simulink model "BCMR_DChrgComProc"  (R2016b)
settings: Solver=FixedStepDiscrete  StartTime=0.0  StopTime=10.0  FixedStep=0.01  RelTol=1e-3  EnableMultiTasking=on
undefined symbols (not defined in the file or in its folder): BCMR_ahBattRatdCpctyBrm_C, BCMR_BattSocErrBsmEna_C, BCMR_eBattRatedEnrgBcp_C, BCMR_G1E0PlatformSwCom_C, BCMR_iMaxChrgCurrPmtdBcp_C, BCMR_numBattTypeBrm_C, BCMR_numComVer2011Brm_C, BCMR_numComVer2015Brm_C, BCMR_tMaxTempPmtdBcp_C, BCMR_uBattRatdPackVoltBcp_C, BCMR_uBattRatdPackVoltBrm_C, BCMR_uMaxChrgCellVoltPmtdBcp_C, BCMR_uMaxPmtDChrgVolt_C
libraries: simulink x32
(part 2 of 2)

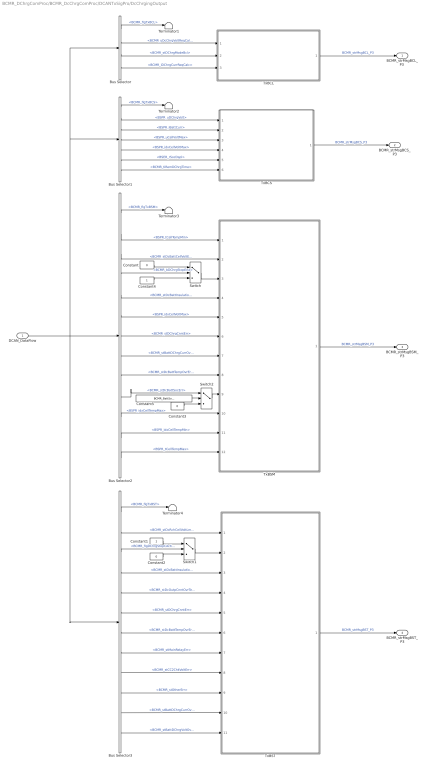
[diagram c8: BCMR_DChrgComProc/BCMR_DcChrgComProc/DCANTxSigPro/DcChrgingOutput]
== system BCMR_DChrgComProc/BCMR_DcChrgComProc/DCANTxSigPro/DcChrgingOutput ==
  DCAN_DataFlow : Inport
  Bus Selector : BusSelector  OutputSignals=BCMR_flgTxBCL,BCMR_uDcChrgVoltReqCalc,BCMR_stDChrgModeBcl,BCMR_iDChrgCurrReqCalc
  Bus Selector1 : BusSelector  OutputSignals=BCMR_flgTxBCS,BSPR_uDChrgVolt,BSPR_iBattCurr,BSPR_uCellVoltMax,BSPR_idxCellVoltMax,BSER_rSocDspl,BCMR_tiRemDChrgTime
  Bus Selector2 : BusSelector  OutputSignals=BCMR_flgTxBSM,BSPR_tCellTempMin,BCMR_stDcBattCellVoltErr,BCMR_bDChrgStopEna,BCMR_stDcBattInsulationErr,BSPR_idxCellVoltMax,BCMR_stDChrgCnntErr,BCMR_stBattDChrgCurrOvrErr,BCMR_stDcBattTempOvrErr,BCMR_stDcBattSocErr,BSPR_idxCellTempMax,BSPR_idxCellTempMin,BSPR_tCellTempMax
  Bus Selector3 : BusSelector  OutputSignals=BCMR_flgTxBST,BCMR_stDcRchCellVoltLmt,BCMR_flgDChrgStopCActive,BCMR_stDcBattInsulationErr,BCMR_stDcOutpCnntOvrTempErr,BCMR_stDChrgCnntErr,BCMR_stDcBattTempOvrErr,BCMR_stMainRelayErr,BCMR_stCC2ChkVoltErr,BCMR_stOtherErr,BCMR_stBattDChrgCurrOvrErr,BCMR_stBattDChrgVoltOvrErr
  Constant : Constant  Value=0  OutDataTypeStr=uint8
  Constant1 : Constant  OutDataTypeStr=uint8
  Constant2 : Constant  Value=0  OutDataTypeStr=uint8
  Constant3 : Constant  Value=0  OutDataTypeStr=uint8
  Constant4 : Constant  OutDataTypeStr=uint8
  Constant5 : Constant  Value=BCMR_BattSocErrBsmEna_C
  Switch : Switch  Criteria=u2 > Threshold  OutDataTypeStr=uint8
  Switch1 : Switch  Criteria=u2 > Threshold  OutDataTypeStr=uint8
  Switch2 : Switch  Criteria=u2 > Threshold  OutDataTypeStr=uint8
  Terminator{1..4} (4 alike) : Terminator
  TxBCL : Subsystem
  TxBCS : Subsystem
  TxBSM : Subsystem
  TxBST : Subsystem
  "BCMR_strMsgBCL_P3 " : Outport  OutDataTypeStr=Bus: MSG_BCL_P3
  BCMR_strMsgBCS_P3 : Outport  Port=2  OutDataTypeStr=Bus: MSG_BCS_P3
  BCMR_strMsgBSM_P3 : Outport  Port=3  OutDataTypeStr=Bus: MSG_BSM_P3
  BCMR_strMsgBST_P3 : Outport  Port=4  OutDataTypeStr=Bus: MSG_BST_P3
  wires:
  TxBCL/1("BCMR_strMsgBCL_P3 ") -> "BCMR_strMsgBCL_P3 "/1  "BCMR_strMsgBCL_P3"
  TxBCS/1(BCMR_strMsgBCS_P3) -> BCMR_strMsgBCS_P3/1  "BCMR_strMsgBCS_P3"
  TxBSM/1(BCMR_strMsgBSM_P3) -> BCMR_strMsgBSM_P3/1  "BCMR_strMsgBSM_P3"
  DCAN_DataFlow/1 -> Bus Selector/1, Bus Selector1/1, Bus Selector3/1, Bus Selector2/1
  Bus Selector2/2 -> TxBSM/1(BCMR_tBattMinTempBsm)  "<BSPR_tCellTempMin>"
  Bus Selector2/3 -> TxBSM/2(BCMR_stBattCellVoltErrBsm)  "<BCMR_stDcBattCellVoltErr>"
  Bus Selector2/5 -> TxBSM/4(BCMR_stBattInsulationErrBsm)  "<BCMR_stDcBattInsulationErr>"
  Bus Selector2/6 -> TxBSM/5(BCMR_numMaxCellVoltAddrBsm)  "<BSPR_idxCellVoltMax>"
  Bus Selector2/7 -> TxBSM/6(BCMR_stBattOutputContErrBsm)  "<BCMR_stDChrgCnntErr>"
  Bus Selector2/8 -> TxBSM/7(BCMR_stBattChrgCurrOvrErrBsm)  "<BCMR_stBattDChrgCurrOvrErr>"
  Bus Selector2/9 -> TxBSM/8(BCMR_stBattTempOvrErrBsm)  "<BCMR_stDcBattTempOvrErr>"
  TxBST/1(BCMR_strMsgBST_P3) -> BCMR_strMsgBST_P3/1  "BCMR_strMsgBST_P3"
  Bus Selector/2 -> TxBCL/1(BCMR_vDcChrgVoltReqBcl)  "<BCMR_uDcChrgVoltReqCalc>"
  Bus Selector/3 -> TxBCL/2(BCMR_stDcChrgModeBcl)  "<BCMR_stDChrgModeBcl>"
  Bus Selector/4 -> TxBCL/3(BCMR_iDcChrgCurrReqBcl)  "<BCMR_iDChrgCurrReqCalc>"
  Bus Selector1/2 -> TxBCS/1(BCMR_vDcChrgVoltReqBcs)  "<BSPR_uDChrgVolt>"
  Bus Selector1/3 -> TxBCS/2(BCMR_iDcChrgCurrReqBcs)  "<BSPR_iBattCurr>"
  Bus Selector1/4 -> TxBCS/3(BCMR_uMaxCellVoltBcs)  "<BSPR_uCellVoltMax>"
  Bus Selector1/5 -> TxBCS/4(BCMR_numMaxCellVoltGrpNumBcs)  "<BSPR_idxCellVoltMax>"
  Bus Selector1/6 -> TxBCS/5(BCMR_rSocDsplBcs)  "<BSER_rSocDspl>"
  Bus Selector1/7 -> TxBCS/6(BCMR_tiDcChrgRemTimeBcs)  "<BCMR_tiRemDChrgTime>"
  Bus Selector2/11 -> TxBSM/10(BCMR_numBattMaxTemptAddrBsm)  "<BSPR_idxCellTempMax>"
  Bus Selector2/12 -> TxBSM/11(BCMR_numBattMinTemptAddrBsm)  "<BSPR_idxCellTempMin>"
  Bus Selector2/13 -> TxBSM/12(BCMR_tBattMaxTempBsm)  "<BSPR_tCellTempMax>"
  Bus Selector3/2 -> TxBST/1(BCMR_stRchCellVoltLmtBst)  "<BCMR_stDcRchCellVoltLmt>"
  Bus Selector3/4 -> TxBST/3(BCMR_stBattInsulationErrBst)  "<BCMR_stDcBattInsulationErr>"
  Bus Selector3/5 -> TxBST/4(BCMR_stOutpCnntOvrTempErrBst)  "<BCMR_stDcOutpCnntOvrTempErr>"
  Bus Selector3/6 -> TxBST/5(BCMR_stChrgCnntErrBst)  "<BCMR_stDChrgCnntErr>"
  Bus Selector3/7 -> TxBST/6(BCMR_stBattOvrTempErrBst)  "<BCMR_stDcBattTempOvrErr>"
  Bus Selector3/8 -> TxBST/7(BCMR_stMainRelayErrBst)  "<BCMR_stMainRelayErr>"
  Bus Selector3/9 -> TxBST/8(BCMR_stCC2ChkVoltErrBst)  "<BCMR_stCC2ChkVoltErr>"
  Bus Selector3/10 -> TxBST/9(BCMR_stOtherErrBst)  "<BCMR_stOtherErr>"
  Bus Selector3/11 -> TxBST/10(BCMR_stChrgCurrAbnrmBst)  "<BCMR_stBattDChrgCurrOvrErr>"
  Bus Selector3/12 -> TxBST/11(BCMR_stChrgVoltAbnrm)  "<BCMR_stBattDChrgVoltOvrErr>"
  Constant/1 -> Switch/1
  Constant4/1 -> Switch/3
  Switch/1 -> TxBSM/3(BCMR_stChrgEnaBsm)
  Bus Selector2/4 -> Switch/2  "<BCMR_bDChrgStopEna>"
  Bus Selector/1 -> Terminator1/1  "<BCMR_flgTxBCL>"
  Bus Selector1/1 -> Terminator2/1  "<BCMR_flgTxBCS>"
  Bus Selector2/1 -> Terminator3/1  "<BCMR_flgTxBSM>"
  Bus Selector3/1 -> Terminator4/1  "<BCMR_flgTxBST>"
  Bus Selector3/3 -> Switch1/2  "<BCMR_flgDChrgStopCActive>"
  Switch1/1 -> TxBST/2(BCMR_stChrgerActStopBst)
  Constant1/1 -> Switch1/1
  Constant2/1 -> Switch1/3
  Constant3/1 -> Switch2/3
  Switch2/1 -> TxBSM/9(BCMR_stBattSocErrBsm)
  Bus Selector2/10 -> Switch2/1  "<BCMR_stDcBattSocErr>"
  Constant5/1 -> Switch2/2

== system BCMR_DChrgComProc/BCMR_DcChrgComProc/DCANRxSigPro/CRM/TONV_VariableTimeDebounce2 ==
  note: Turn On Delay Time Deboune
  u : Inport
  T : Inport  Port=2
  dT : Inport  Port=3
  Add : Sum
  Constant1 : Constant  Value=0  OutDataTypeStr=single
  Constant2 : Constant  OutDataTypeStr=uint8
  Constant3 : Constant  Value=0  OutDataTypeStr=uint8
  Delay : Delay  DelayLength=1  InitialCondition=0
  MinMax : MinMax  Inputs=2
  Product : Product  OutMin=[0]  OutMax=[65535]  OutDataTypeStr=single
  Relational Operator : RelationalOperator  Operator=>  OutDataTypeStr=boolean  RndMeth=Simplest
  Switch : Switch  Criteria=u2 ~= 0
  Switch1 : Switch  Criteria=u2 ~= 0
  y : Outport
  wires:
  Switch1/1 -> Product/1
  Constant3/1 -> Switch1/3
  Constant2/1 -> Switch1/1
  u/1 -> Switch1/2, Switch/2
  dT/1 -> Switch/1
  Constant1/1 -> Switch/3
  Add/1 -> Product/2
  Product/1 -> Relational Operator/1, Delay/1
  Switch/1 -> Add/1
  Delay/1 -> MinMax/2
  Relational Operator/1 -> y/1
  T/1 -> MinMax/1, Relational Operator/2
  MinMax/1 -> Add/2

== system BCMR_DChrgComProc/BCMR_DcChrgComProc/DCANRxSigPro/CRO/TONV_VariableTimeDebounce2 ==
  note: Turn On Delay Time Deboune
  u : Inport
  T : Inport  Port=2
  dT : Inport  Port=3
  Add : Sum
  Constant1 : Constant  Value=0  OutDataTypeStr=single
  Constant2 : Constant  OutDataTypeStr=uint8
  Constant3 : Constant  Value=0  OutDataTypeStr=uint8
  Delay : Delay  DelayLength=1  InitialCondition=0
  MinMax : MinMax  Inputs=2
  Product : Product  OutMin=[0]  OutMax=[65535]  OutDataTypeStr=single
  Relational Operator : RelationalOperator  Operator=>  OutDataTypeStr=boolean  RndMeth=Simplest
  Switch : Switch  Criteria=u2 ~= 0
  Switch1 : Switch  Criteria=u2 ~= 0
  y : Outport
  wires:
  Switch1/1 -> Product/1
  Constant3/1 -> Switch1/3
  Constant2/1 -> Switch1/1
  u/1 -> Switch1/2, Switch/2
  dT/1 -> Switch/1
  Constant1/1 -> Switch/3
  Add/1 -> Product/2
  Product/1 -> Relational Operator/1, Delay/1
  Switch/1 -> Add/1
  Delay/1 -> MinMax/2
  Relational Operator/1 -> y/1
  T/1 -> MinMax/1, Relational Operator/2
  MinMax/1 -> Add/2

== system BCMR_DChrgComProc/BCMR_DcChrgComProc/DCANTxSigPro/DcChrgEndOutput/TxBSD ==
  BCMR_tBattMaxTempBsd : Inport
  BCMR_tBattMinTempBsd : Inport  Port=2
  BCMR_vBattMinCellVoltBsd : Inport  Port=3
  BCMR_vBattMaxCellVoltBsd : Inport  Port=4
  BCMR_rBattSocBsd : Inport  Port=5
  Bus Creator : BusCreator  Inputs=5  OutDataTypeStr=Bus: MSG_BSD_P4
  "BCMR_strMsgBSD_P4 " : Outport  OutDataTypeStr=Bus: MSG_BSD_P4
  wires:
  BCMR_tBattMaxTempBsd/1 -> Bus Creator/1
  BCMR_tBattMinTempBsd/1 -> Bus Creator/2
  BCMR_vBattMinCellVoltBsd/1 -> Bus Creator/3
  BCMR_vBattMaxCellVoltBsd/1 -> Bus Creator/4
  BCMR_rBattSocBsd/1 -> Bus Creator/5
  Bus Creator/1 -> "BCMR_strMsgBSD_P4 "/1

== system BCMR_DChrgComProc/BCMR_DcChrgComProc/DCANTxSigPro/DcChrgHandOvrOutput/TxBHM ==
  Bus Creator : BusCreator  Inputs=1  OutDataTypeStr=Bus: MSG_BHM_P1
  Constant : Constant  Value=BCMR_uMaxPmtDChrgVolt_C
  "BCMR_strMsgBHM_P1 " : Outport  OutDataTypeStr=Bus: MSG_BHM_P1  InitialOutput=[421.8]
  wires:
  Bus Creator/1 -> "BCMR_strMsgBHM_P1 "/1  "BCMR_strMsgBHM_P1"
  Constant/1 -> Bus Creator/1

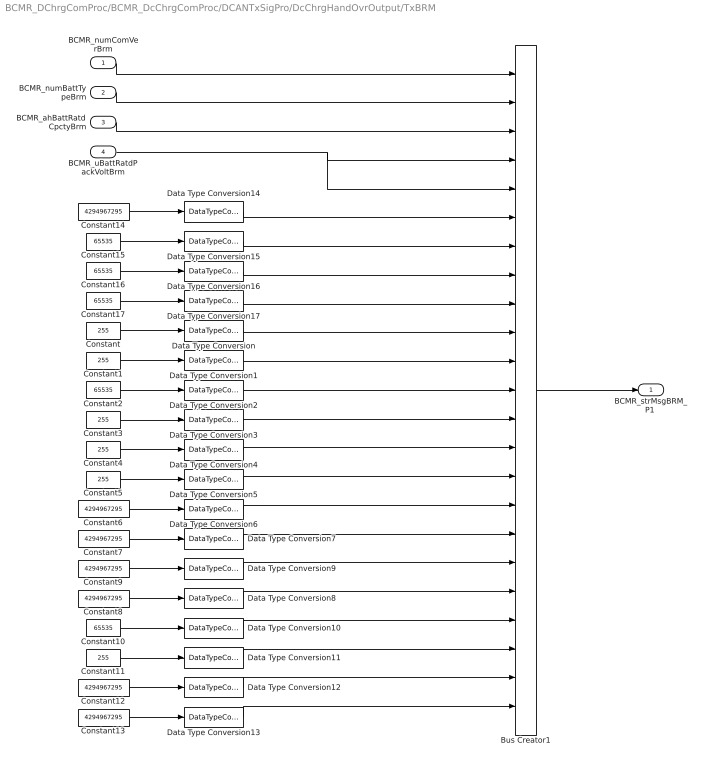
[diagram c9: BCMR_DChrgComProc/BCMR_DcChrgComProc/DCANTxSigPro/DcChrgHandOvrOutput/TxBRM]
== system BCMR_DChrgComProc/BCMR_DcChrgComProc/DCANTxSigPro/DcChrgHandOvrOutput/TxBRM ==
  BCMR_numComVerBrm : Inport
  BCMR_numBattTypeBrm : Inport  Port=2
  BCMR_ahBattRatdCpctyBrm : Inport  Port=3
  BCMR_uBattRatdPackVoltBrm : Inport  Port=4
  Bus Creator1 : BusCreator  Inputs=23  OutDataTypeStr=Bus: MSG_BRM_P1
  Constant{,1,3..5,11} (6 alike) : Constant  Value=255
  Constant{2,10,15..17} (5 alike) : Constant  Value=65535
  Constant{6..9,12..14} (7 alike) : Constant  Value=4294967295
  Data Type Conversion{,1,3..5,11} (6 alike) : DataTypeConversion  OutDataTypeStr=uint8
  Data Type Conversion{2,10,15..17} (5 alike) : DataTypeConversion  OutDataTypeStr=uint16
  Data Type Conversion{6..9,12..14} (7 alike) : DataTypeConversion  OutDataTypeStr=uint32
  "BCMR_strMsgBRM_P1 " : Outport  OutDataTypeStr=Bus: MSG_BRM_P1
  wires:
  BCMR_numBattTypeBrm/1 -> Bus Creator1/2
  BCMR_ahBattRatdCpctyBrm/1 -> Bus Creator1/3
  BCMR_numComVerBrm/1 -> Bus Creator1/1
  Bus Creator1/1 -> "BCMR_strMsgBRM_P1 "/1
  Constant/1 -> Data Type Conversion/1
  Constant1/1 -> Data Type Conversion1/1
  Constant2/1 -> Data Type Conversion2/1
  Constant3/1 -> Data Type Conversion3/1
  Constant4/1 -> Data Type Conversion4/1
  Constant5/1 -> Data Type Conversion5/1
  Constant6/1 -> Data Type Conversion6/1
  Constant7/1 -> Data Type Conversion7/1
  Constant8/1 -> Data Type Conversion8/1
  Constant9/1 -> Data Type Conversion9/1
  Constant10/1 -> Data Type Conversion10/1
  Constant11/1 -> Data Type Conversion11/1
  Constant12/1 -> Data Type Conversion12/1
  Constant13/1 -> Data Type Conversion13/1
  Data Type Conversion13/1 -> Bus Creator1/23
  Data Type Conversion/1 -> Bus Creator1/10
  Data Type Conversion1/1 -> Bus Creator1/11
  Data Type Conversion2/1 -> Bus Creator1/12
  Data Type Conversion3/1 -> Bus Creator1/13
  Data Type Conversion4/1 -> Bus Creator1/14
  Data Type Conversion5/1 -> Bus Creator1/15
  Data Type Conversion6/1 -> Bus Creator1/16
  Data Type Conversion7/1 -> Bus Creator1/17
  Data Type Conversion9/1 -> Bus Creator1/18
  Data Type Conversion8/1 -> Bus Creator1/19
  Data Type Conversion10/1 -> Bus Creator1/20
  Data Type Conversion11/1 -> Bus Creator1/21
  Data Type Conversion12/1 -> Bus Creator1/22
  Constant14/1 -> Data Type Conversion14/1
  Constant15/1 -> Data Type Conversion15/1
  Constant16/1 -> Data Type Conversion16/1
  Constant17/1 -> Data Type Conversion17/1
  Data Type Conversion17/1 -> Bus Creator1/9
  Data Type Conversion14/1 -> Bus Creator1/6
  Data Type Conversion15/1 -> Bus Creator1/7
  Data Type Conversion16/1 -> Bus Creator1/8
  BCMR_uBattRatdPackVoltBrm/1 -> Bus Creator1/5, Bus Creator1/4

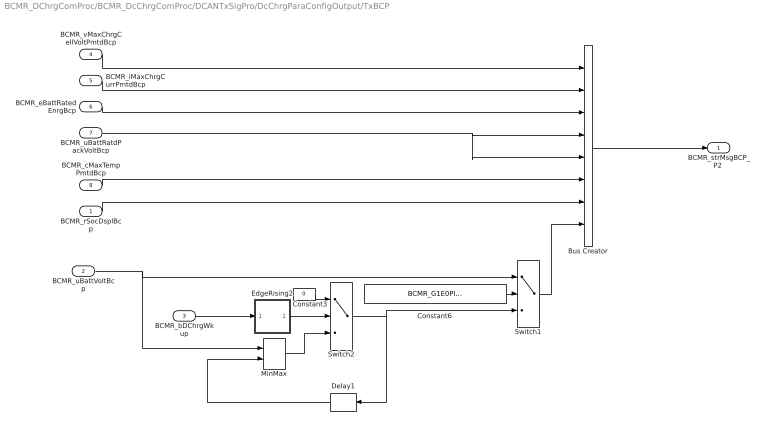
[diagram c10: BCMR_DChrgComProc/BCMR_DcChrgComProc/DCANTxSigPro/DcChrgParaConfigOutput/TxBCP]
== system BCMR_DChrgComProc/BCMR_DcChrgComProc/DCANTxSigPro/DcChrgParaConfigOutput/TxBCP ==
  BCMR_rSocDsplBcp : Inport
  BCMR_uBattVoltBcp : Inport  Port=2
  BCMR_bDChrgWkup : Inport  Port=3
  BCMR_vMaxChrgCellVoltPmtdBcp : Inport  Port=4
  BCMR_iMaxChrgCurrPmtdBcp : Inport  Port=5
  BCMR_eBattRatedEnrgBcp : Inport  Port=6
  BCMR_uBattRatdPackVoltBcp : Inport  Port=7
  BCMR_cMaxTempPmtdBcp : Inport  Port=8
  Bus Creator : BusCreator  Inputs=8  OutDataTypeStr=Bus: MSG_BCP_P2
  Constant3 : Constant  Value=0  OutDataTypeStr=single
  Constant6 : Constant  Value=BCMR_G1E0PlatformSwCom_C
  Delay1 : Delay  DelayLength=1  InitialCondition=0
  EdgeRising2 : Subsystem  TreatAsAtomicUnit=on  RTWFcnName=EdgeRising  RTWFileName=SrvLib
  MinMax : MinMax  Function=max  Inputs=2
  Switch1 : Switch  Criteria=u2 ~= 0
  Switch2 : Switch  Criteria=u2 ~= 0
  "BCMR_strMsgBCP_P2 " : Outport  OutDataTypeStr=Bus: MSG_BCP_P2
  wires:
  BCMR_vMaxChrgCellVoltPmtdBcp/1 -> Bus Creator/1
  BCMR_iMaxChrgCurrPmtdBcp/1 -> Bus Creator/2
  BCMR_eBattRatedEnrgBcp/1 -> Bus Creator/3
  Bus Creator/1 -> "BCMR_strMsgBCP_P2 "/1
  BCMR_rSocDsplBcp/1 -> Bus Creator/7
  BCMR_cMaxTempPmtdBcp/1 -> Bus Creator/6
  BCMR_uBattRatdPackVoltBcp/1 -> Bus Creator/5, Bus Creator/4
  BCMR_bDChrgWkup/1 -> EdgeRising2/1(u)
  EdgeRising2/1(y) -> Switch2/2
  Constant3/1 -> Switch2/1
  Switch2/1 -> Delay1/1, Switch1/3
  MinMax/1 -> Switch2/3
  Delay1/1 -> MinMax/2
  Switch1/1 -> Bus Creator/8
  BCMR_uBattVoltBcp/1 -> Switch1/1, MinMax/1
  Constant6/1 -> Switch1/2

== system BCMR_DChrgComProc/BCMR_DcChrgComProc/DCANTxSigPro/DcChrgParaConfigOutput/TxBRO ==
  BCMR_stBmsRdyBro : Inport
  Bus Creator1 : BusCreator  Inputs=1  OutDataTypeStr=Bus: MSG_BRO_P2
  BCMR_strMsgBRO_P2 : Outport  OutDataTypeStr=Bus: MSG_BRO_P2
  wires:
  BCMR_stBmsRdyBro/1 -> Bus Creator1/1
  Bus Creator1/1 -> BCMR_strMsgBRO_P2/1

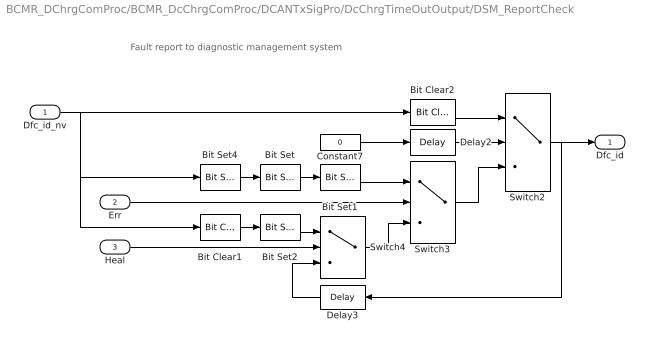
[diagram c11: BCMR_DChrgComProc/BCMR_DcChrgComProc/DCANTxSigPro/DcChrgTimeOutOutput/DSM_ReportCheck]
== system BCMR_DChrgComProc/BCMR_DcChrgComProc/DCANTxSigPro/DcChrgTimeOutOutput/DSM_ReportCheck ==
  note: Fault report to diagnostic management system
  Dfc_id_nv : Inport  OutDataTypeStr=uint8
  Err : Inport  Port=2
  Heal : Inport  Port=3
  Bit Clear1 : simulink/Logic and Bit Operations/Bit Clear  iBit=4
  Bit Clear2 : simulink/Logic and Bit Operations/Bit Clear  iBit=3
  Bit Set : simulink/Logic and Bit Operations/Bit Set  iBit=4
  Bit Set1 : simulink/Logic and Bit Operations/Bit Set  iBit=3
  Bit Set2 : simulink/Logic and Bit Operations/Bit Set  iBit=3
  Bit Set4 : simulink/Logic and Bit Operations/Bit Set  iBit=7
  Constant7 : Constant  Value=0  OutDataTypeStr=boolean
  Delay2 : Delay  DelayLength=1  InitialCondition=1
  Delay3 : Delay  DelayLength=1  InitialCondition=0
  Switch2 : Switch  Criteria=u2 ~= 0
  Switch3 : Switch  Criteria=u2 ~= 0
  Switch4 : Switch  Criteria=u2 ~= 0
  Dfc_id : Outport  OutDataTypeStr=uint8
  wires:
  Dfc_id_nv/1 -> Bit Clear2/1, Bit Set4/1, Bit Clear1/1
  Bit Set4/1 -> Bit Set/1
  Constant7/1 -> Delay2/1
  Delay2/1 -> Switch2/2
  Switch3/1 -> Switch2/3
  Bit Clear2/1 -> Switch2/1
  Switch2/1 -> Delay3/1, Dfc_id/1
  Bit Set1/1 -> Switch3/1
  Bit Set/1 -> Bit Set1/1
  Switch4/1 -> Switch3/3
  Err/1 -> Switch3/2
  Bit Set2/1 -> Switch4/1
  Bit Clear1/1 -> Bit Set2/1
  Delay3/1 -> Switch4/3
  Heal/1 -> Switch4/2

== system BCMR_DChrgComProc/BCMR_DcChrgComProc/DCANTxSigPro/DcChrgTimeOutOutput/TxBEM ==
  BCMR_stSpn3901TimeoutBem : Inport
  BCMR_stSpn3902TimeoutBem : Inport  Port=2
  BCMR_stSpn3903TimeoutBem : Inport  Port=3
  BCMR_stSpn3904TimeoutBem : Inport  Port=4
  BCMR_stSpn3905TimeoutBem : Inport  Port=5
  BCMR_stSpn3906TimeoutBem : Inport  Port=6
  BCMR_stSpn3907TimeoutBem : Inport  Port=7
  BCMR_stOtherErrBem : Inport  Port=8
  Bus Creator : BusCreator  Inputs=8  OutDataTypeStr=Bus: MSG_BEM_ERR
  "BCMR_strMsgBEM_ERR " : Outport  OutDataTypeStr=Bus: MSG_BEM_ERR
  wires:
  Bus Creator/1 -> "BCMR_strMsgBEM_ERR "/1
  BCMR_stSpn3901TimeoutBem/1 -> Bus Creator/1
  BCMR_stSpn3902TimeoutBem/1 -> Bus Creator/2
  BCMR_stSpn3903TimeoutBem/1 -> Bus Creator/3
  BCMR_stSpn3904TimeoutBem/1 -> Bus Creator/4
  BCMR_stSpn3905TimeoutBem/1 -> Bus Creator/5
  BCMR_stSpn3906TimeoutBem/1 -> Bus Creator/6
  BCMR_stSpn3907TimeoutBem/1 -> Bus Creator/7
  BCMR_stOtherErrBem/1 -> Bus Creator/8

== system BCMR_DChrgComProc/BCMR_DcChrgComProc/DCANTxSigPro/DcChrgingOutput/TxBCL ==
  BCMR_vDcChrgVoltReqBcl : Inport
  BCMR_stDcChrgModeBcl : Inport  Port=2
  BCMR_iDcChrgCurrReqBcl : Inport  Port=3
  Bus Creator : BusCreator  Inputs=3  OutDataTypeStr=Bus: MSG_BCL_P3
  Gain : Gain  Gain=-1
  "BCMR_strMsgBCL_P3 " : Outport  OutDataTypeStr=Bus: MSG_BCL_P3
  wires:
  Bus Creator/1 -> "BCMR_strMsgBCL_P3 "/1
  BCMR_iDcChrgCurrReqBcl/1 -> Gain/1
  BCMR_stDcChrgModeBcl/1 -> Bus Creator/2
  BCMR_vDcChrgVoltReqBcl/1 -> Bus Creator/1
  Gain/1 -> Bus Creator/3

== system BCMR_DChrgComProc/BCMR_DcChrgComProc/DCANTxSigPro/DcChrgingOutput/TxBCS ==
  BCMR_vDcChrgVoltReqBcs : Inport
  BCMR_iDcChrgCurrReqBcs : Inport  Port=2
  BCMR_uMaxCellVoltBcs : Inport  Port=3
  BCMR_numMaxCellVoltGrpNumBcs : Inport  Port=4
  BCMR_rSocDsplBcs : Inport  Port=5
  BCMR_tiDcChrgRemTimeBcs : Inport  Port=6
  Bus Creator1 : BusCreator  Inputs=6  OutDataTypeStr=Bus: MSG_BCS_P3
  Data Type Conversion : DataTypeConversion  OutDataTypeStr=uint8
  Data Type Conversion1 : DataTypeConversion  OutDataTypeStr=uint16
  BCMR_strMsgBCS_P3 : Outport  OutDataTypeStr=Bus: MSG_BCS_P3
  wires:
  BCMR_numMaxCellVoltGrpNumBcs/1 -> Bus Creator1/4
  BCMR_uMaxCellVoltBcs/1 -> Bus Creator1/3
  BCMR_iDcChrgCurrReqBcs/1 -> Bus Creator1/2
  BCMR_vDcChrgVoltReqBcs/1 -> Bus Creator1/1
  BCMR_tiDcChrgRemTimeBcs/1 -> Data Type Conversion1/1
  Data Type Conversion/1 -> Bus Creator1/5
  Data Type Conversion1/1 -> Bus Creator1/6
  Bus Creator1/1 -> BCMR_strMsgBCS_P3/1
  BCMR_rSocDsplBcs/1 -> Data Type Conversion/1

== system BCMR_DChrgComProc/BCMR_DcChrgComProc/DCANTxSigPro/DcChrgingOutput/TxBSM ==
  BCMR_tBattMinTempBsm : Inport
  BCMR_stBattCellVoltErrBsm : Inport  Port=2
  BCMR_stChrgEnaBsm : Inport  Port=3
  BCMR_stBattInsulationErrBsm : Inport  Port=4
  BCMR_numMaxCellVoltAddrBsm : Inport  Port=5
  BCMR_stBattOutputContErrBsm : Inport  Port=6
  BCMR_stBattChrgCurrOvrErrBsm : Inport  Port=7
  BCMR_stBattTempOvrErrBsm : Inport  Port=8
  BCMR_stBattSocErrBsm : Inport  Port=9
  BCMR_numBattMaxTemptAddrBsm : Inport  Port=10
  BCMR_numBattMinTemptAddrBsm : Inport  Port=11
  BCMR_tBattMaxTempBsm : Inport  Port=12
  Bus Creator2 : BusCreator  Inputs=12  OutDataTypeStr=Bus: MSG_BSM_P3
  BCMR_strMsgBSM_P3 : Outport  OutDataTypeStr=Bus: MSG_BSM_P3
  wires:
  BCMR_stBattTempOvrErrBsm/1 -> Bus Creator2/8
  BCMR_stBattChrgCurrOvrErrBsm/1 -> Bus Creator2/7
  BCMR_stBattOutputContErrBsm/1 -> Bus Creator2/6
  BCMR_numMaxCellVoltAddrBsm/1 -> Bus Creator2/5
  BCMR_stBattInsulationErrBsm/1 -> Bus Creator2/4
  BCMR_stBattCellVoltErrBsm/1 -> Bus Creator2/2
  BCMR_tBattMinTempBsm/1 -> Bus Creator2/1
  BCMR_stBattSocErrBsm/1 -> Bus Creator2/9
  BCMR_numBattMaxTemptAddrBsm/1 -> Bus Creator2/10
  BCMR_numBattMinTemptAddrBsm/1 -> Bus Creator2/11
  BCMR_tBattMaxTempBsm/1 -> Bus Creator2/12
  BCMR_stChrgEnaBsm/1 -> Bus Creator2/3
  Bus Creator2/1 -> BCMR_strMsgBSM_P3/1

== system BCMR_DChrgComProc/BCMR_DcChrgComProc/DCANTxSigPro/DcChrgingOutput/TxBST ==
  BCMR_stRchCellVoltLmtBst : Inport
  BCMR_stChrgerActStopBst : Inport  Port=2
  BCMR_stBattInsulationErrBst : Inport  Port=3
  BCMR_stOutpCnntOvrTempErrBst : Inport  Port=4
  BCMR_stChrgCnntErrBst : Inport  Port=5
  BCMR_stBattOvrTempErrBst : Inport  Port=6
  BCMR_stMainRelayErrBst : Inport  Port=7
  BCMR_stCC2ChkVoltErrBst : Inport  Port=8
  BCMR_stOtherErrBst : Inport  Port=9
  BCMR_stChrgCurrAbnrmBst : Inport  Port=10
  BCMR_stChrgVoltAbnrm : Inport  Port=11
  Bus Creator3 : BusCreator  Inputs=14  OutDataTypeStr=Bus: MSG_BST_P3
  Constant : Constant  Value=0  OutDataTypeStr=uint8
  BCMR_strMsgBST_P3 : Outport  OutDataTypeStr=Bus: MSG_BST_P3
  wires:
  Constant/1 -> Bus Creator3/7
  BCMR_stOutpCnntOvrTempErrBst/1 -> Bus Creator3/6
  BCMR_stBattInsulationErrBst/1 -> Bus Creator3/5
  BCMR_stChrgerActStopBst/1 -> Bus Creator3/4
  BCMR_stRchCellVoltLmtBst/1 -> Bus Creator3/1, Bus Creator3/2, Bus Creator3/3
  Bus Creator3/1 -> BCMR_strMsgBST_P3/1
  BCMR_stChrgCnntErrBst/1 -> Bus Creator3/8
  BCMR_stBattOvrTempErrBst/1 -> Bus Creator3/9
  BCMR_stMainRelayErrBst/1 -> Bus Creator3/10
  BCMR_stCC2ChkVoltErrBst/1 -> Bus Creator3/11
  BCMR_stOtherErrBst/1 -> Bus Creator3/12
  BCMR_stChrgCurrAbnrmBst/1 -> Bus Creator3/13
  BCMR_stChrgVoltAbnrm/1 -> Bus Creator3/14

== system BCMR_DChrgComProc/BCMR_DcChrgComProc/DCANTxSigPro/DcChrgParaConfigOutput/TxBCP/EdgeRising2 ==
  u : Inport
  Delay1 : Delay  DelayLength=1  InitialCondition=1
  Logical Operator3 : Logic  Operator=NOT  AllPortsSameDT=off  OutDataTypeStr=boolean
  Logical Operator4 : Logic  AllPortsSameDT=off  OutDataTypeStr=boolean
  y : Outport
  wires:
  Logical Operator4/1 -> y/1
  Logical Operator3/1 -> Logical Operator4/1
  u/1 -> Delay1/1, Logical Operator4/2
  Delay1/1 -> Logical Operator3/1
